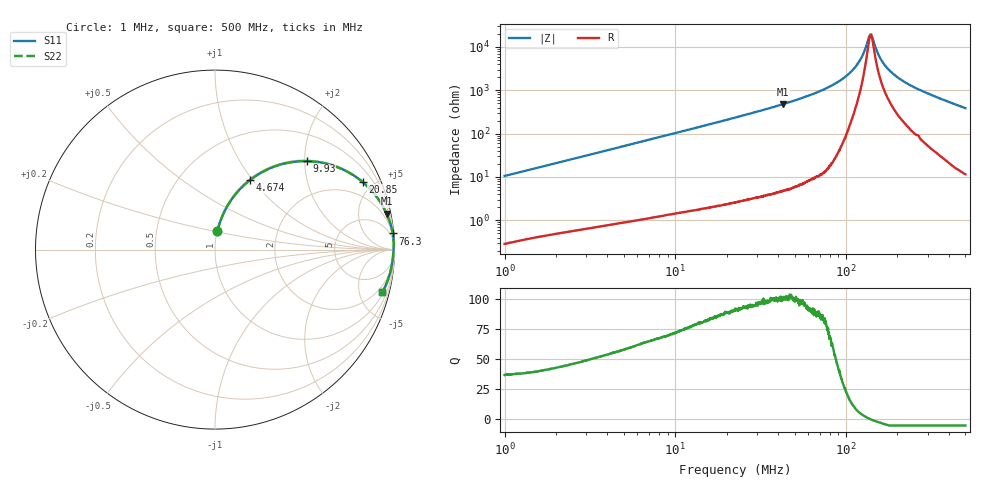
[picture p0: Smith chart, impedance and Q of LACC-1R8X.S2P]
!s-Parameter Generated by FASTRON Sdn. Bhd.
!FASTRON P/N : LACC-1R8X
!Keysight Technologies,E4991B,MY54100416,A.01.15
!Date: Wed Mar 18 09:02:33 2026
!Version  : Rev00 Wed Mar 18 09:02:33 2026
!Data & Calibration Information:
!PortZ  Port1:50+j0  Port2:50+j0
!When reading, reference impedance value at option line is always used.
!Remarks : This data is being provided solely for informational purposes.
!Freq	S11	S21	S12	S22
# Hz S dB R 50
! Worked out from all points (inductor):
!   1601 points, 1 MHz to 500 MHz, reference 50 ohm
!   read as one part in series: L = 1.67 uH near 1.032 MHz
!   highest Q = 101 at 42.77 MHz (marker M1), where L = 1.78 uH
!   self-resonance near 139.3 MHz
!   S11 on the Smith chart (normalised r, x): 1 MHz: 1.01, +0.21; 4.674 MHz: 1.02, +0.96; 9.93 MHz: 1.03, +2.04; 20.85 MHz: 1.05, +4.34; 76.3 MHz: 1, +22; 500 MHz: 1.23, -7.73
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1000000  -19.61 82.4  -0.07 -6.0  -0.07 -6.0  -19.61 82.4
2820919  -11.08 72.6  -0.41 -16.2  -0.41 -16.2  -11.08 72.6
4673927  -7.30 63.4  -0.97 -25.5  -0.97 -25.5  -7.30 63.4
7957584  -4.03 50.2  -2.29 -39.0  -2.29 -39.0  -4.03 50.2
9929607  -2.98 44.0  -3.16 -45.2  -3.16 -45.2  -2.98 44.0
2.085075e7  -0.87 24.6  -7.61 -64.7  -7.61 -64.7  -0.87 24.6
2.236068e7  -0.77 23.1  -8.13 -66.3  -8.13 -66.3  -0.77 23.1
4.2775e7  -0.20 11.8  -13.80 -77.6  -13.80 -77.6  -0.20 11.8
6.307767e7  -0.08 7.1  -18.16 -82.3  -18.16 -82.3  -0.08 7.1
7.630124e7  -0.05 5.2  -20.89 -84.1  -20.89 -84.1  -0.05 5.2
9.520996e7  -0.03 3.1  -25.25 -85.0  -25.25 -85.0  -0.03 3.1
1.116461e8  -0.03 1.8  -30.18 -82.7  -30.18 -82.7  -0.03 1.8
1.235099e8  -0.04 1.0  -35.32 -75.5  -35.32 -75.5  -0.04 1.0
1.355771e8  -0.04 0.2  -44.08 -39.2  -44.08 -39.2  -0.04 0.2
1.387738e8  -0.04 0.0  -45.75 -8.8  -45.75 -8.8  -0.04 0.0
1.425987e8  -0.05 -0.2  -44.44 27.5  -44.44 27.5  -0.05 -0.2
1.517418e8  -0.05 -0.6  -38.05 62.0  -38.05 62.0  -0.05 -0.6
1.589818e8  -0.05 -1.0  -34.71 69.9  -34.71 69.9  -0.05 -1.0
1.77937e8  -0.06 -1.9  -29.55 76.7  -29.55 76.7  -0.06 -1.9
2.070397e8  -0.07 -3.1  -25.24 79.6  -25.24 79.6  -0.07 -3.1
2.543648e8  -0.10 -5.0  -21.21 80.2  -21.21 80.2  -0.10 -5.0
5e8  -0.34 -14.4  -12.09 73.9  -12.09 73.9  -0.34 -14.4
